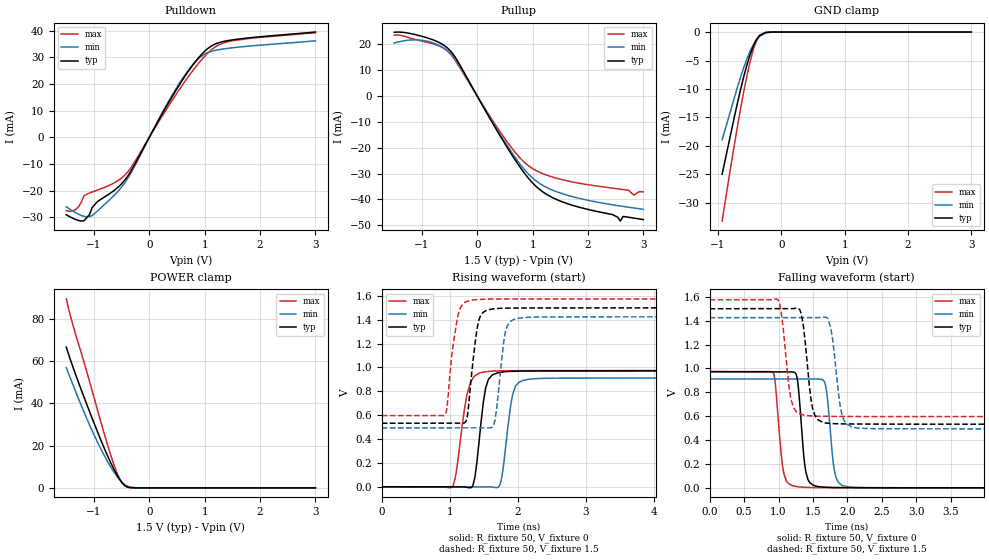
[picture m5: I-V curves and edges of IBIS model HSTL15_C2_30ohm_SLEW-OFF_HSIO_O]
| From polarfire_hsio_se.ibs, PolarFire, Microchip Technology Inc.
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|   Model HSTL15_C2_30ohm_SLEW-OFF_HSIO_O
[Model]   HSTL15_C2_30ohm_SLEW-OFF_HSIO_O
Model_type   Output
Polarity   Non-Inverting
Enable   Active-High
Vmeas =   0.75
Cref =   5p
Rref =   50
Vref =   0.75
|   typ   min   max
C_comp_pullup   1.335e-12   1.335e-12   1.380e-12
C_comp_pulldown  1.335e-12   1.335e-12   1.380e-12
[Temperature Range]  25C   100C   -40C
[Voltage Range]  1.5   1.425   1.575
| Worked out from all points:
|   slope of the pulldown table from 0 to 0.225 V, typ, clamps not added: 26.4 ohm
|   slope of the pullup table from 0 to 0.225 V, typ, clamps not added: 26.4 ohm
|   GND clamp passes 1 mA (typ) near -0.37 V on its own axis
|   POWER clamp passes 1 mA (typ) near -0.43 V on its own axis
|   rising waveform, R_fixture 50, V_fixture 0: 20-80 % time 117ps typ, 120ps min, 143ps max; typ from 0 V to 0.972 V
|   rising waveform, R_fixture 50, V_fixture 1.5: 20-80 % time 111ps typ, 107ps min, 121ps max; typ from 0.533 V to 1.5 V
|   falling waveform, R_fixture 50, V_fixture 0: 20-80 % time 83.1ps typ, 87.6ps min, 88.6ps max; typ from 0.972 V to 0 V
|   falling waveform, R_fixture 50, V_fixture 1.5: 20-80 % time 105ps typ, 112ps min, 108ps max; typ from 1.5 V to 0.533 V
[GND Clamp]
| Voltage   I(typ)   I(min)   I(max)
-935.2mV  -24.96mA   -18.92mA   -33.17mA
-738.3mV  -14.72mA   -11.38mA   -19.54mA
-639.8mV  -9.903mA   -7.788mA   -13.22mA
-590.6mV  -7.7mA     -6.143mA   -10.29mA
-541.4mV  -5.692mA   -4.645mA   -7.577mA
-492.2mV  -3.93mA    -3.33mA    -5.153mA
-443mV    -2.467mA   -2.229mA   -3.103mA
-393.7mV  -1.355mA   -1.366mA   -1.54mA
-344.5mV  -621.9uA   -750.5uA   -567.2uA
-246.1mV  -72.57uA   -154.2uA   -30.93uA
-147.7mV  -5.325uA   -20.63uA   -1.146uA
3V        0A         0A         0A
[POWER Clamp]
| Voltage   I(typ)   I(min)   I(max)
-1.5V     66.64mA    56.9mA     89.46mA
-1.427V   60.81mA    51.96mA    81.57mA
-1.329V   53.43mA    45.4mA     72.34mA
-1.083V   36.31mA    29.95mA    50.59mA
-885.9mV  23.26mA    18.98mA    32.15mA
-738.3mV  14.22mA    11.74mA    18.91mA
-590.6mV  6.331mA    5.649mA    7.47mA
-492.2mV  2.418mA    2.54mA     2.302mA
-443mV    1.134mA    1.422mA    896.4uA
-344.5mV  93.53uA    323uA      39.71uA
-246.1mV  3.484uA    76.21uA    1.36uA
3V        0A         0A         0A
[Pullup]
| Voltage   I(typ)   I(min)   I(max)
-1.5V     24.72mA    20.6mA     23.64mA
-935.2mV  22.77mA    21.42mA    21mA
-492.2mV  17.69mA    16.75mA    16.47mA
609.4mV   -22.23mA   -21.4mA    -19.75mA
890.6mV   -30.94mA   -29.43mA   -26.4mA
1.172V    -36.92mA   -34.44mA   -29.95mA
1.746V    -42.48mA   -39.12mA   -33.38mA
2.435V    -45.85mA   -42.09mA   -35.65mA
2.583V    -48.4mA    -42.58mA   -36.06mA
2.632V    -46.65mA   -42.73mA   -36.2mA
2.829V    -47.27mA   -43.35mA   -38.35mA
3V        -47.83mA   -43.86mA   -37.12mA
[Pulldown]
| Voltage   I(typ)   I(min)   I(max)
-1.5V     -29.1mA    -26.11mA   -27.59mA
-1.329V   -30.88mA   -28.35mA   -27.03mA
-1.23V    -31.45mA   -29.34mA   -24.49mA
-1.083V   -29.08mA   -29.8mA    -20.97mA
-935.2mV  -24.11mA   -27.7mA    -19.8mA
-590.6mV  -19.21mA   -20.85mA   -16.61mA
-344.5mV  -13.14mA   -13.83mA   -11.81mA
562.5mV   20.33mA    20.9mA     18.56mA
843.8mV   28.69mA    28.63mA    26.59mA
1.078V    33.68mA    31.99mA    32.03mA
1.5V      36.55mA    33.59mA    36.2mA
3V        39.5mA     36.21mA    39.23mA
[Ramp]
dV/dt_r   0.583141/0.116851n  0.547234/0.119678n  0.584778/0.143443n
dV/dt_f   0.580324/0.105261n  0.5588/0.111658n  0.587212/0.107647n
R_load = 50
[Rising Waveform]
R_fixture = 50
V_fixture = 0
V_fixture_min = 0
V_fixture_max = 0
| Time   V(typ)   V(min)   V(max)
0s        1.583uV    1.672uV    2.452uV
1.032ns   -626.1uV   -570.8uV   -4.18mV
1.252ns   -4.816mV   -692.8uV   772.9mV
1.314ns   -7.293mV   -727.2uV   886.8mV
1.369ns   82.19mV    -757.7uV   931mV
1.523ns   816.3mV    -843.2uV   964.2mV
1.735ns   958.4mV    15.77mV    971.7mV
1.922ns   967.9mV    770.4mV    973mV
2.147ns   970.2mV    900mV      973.6mV
10ns      971.9mV    912.1mV    974.6mV
[Rising Waveform]
R_fixture = 50
V_fixture = 1.5
V_fixture_min = 1.425
V_fixture_max = 1.575
| Time   V(typ)   V(min)   V(max)
0s        532.8mV    493.6mV    596.3mV
929ps     533.3mV    494.1mV    604.2mV
1.122ns   533.4mV    494.1mV    1.442V
1.248ns   568.1mV    494.2mV    1.552V
1.309ns   879.4mV    494.2mV    1.563V
1.448ns   1.43V      494.3mV    1.571V
1.65ns    1.492V     528.2mV    1.573V
1.815ns   1.497V     1.296V     1.574V
2.024ns   1.498V     1.414V     1.574V
10ns      1.5V       1.425V     1.575V
[Falling Waveform]
R_fixture = 50
V_fixture = 0
V_fixture_min = 0
V_fixture_max = 0
| Time   V(typ)   V(min)   V(max)
0s        971.9mV    912.1mV    974.7mV
924ps     971.2mV    911.5mV    961.1mV
1.078ns   971.1mV    911.4mV    117.9mV
1.26ns    943.6mV    911.3mV    10.78mV
1.396ns   135.9mV    911.2mV    4.517mV
1.577ns   10.8mV     911.1mV    2.071mV
1.698ns   5.016mV    807.1mV    1.534mV
1.834ns   2.412mV    88.43mV    1.28mV
2.013ns   1.487mV    8.407mV    945.2uV
10ns      2.616uV    2.733uV    3.343uV
[Falling Waveform]
R_fixture = 50
V_fixture = 1.5
V_fixture_min = 1.425
V_fixture_max = 1.575
| Time   V(typ)   V(min)   V(max)
0s        1.5V       1.425V     1.575V
994ps     1.501V     1.426V     1.574V
1.18ns    1.501V     1.426V     742.4mV
1.308ns   1.492V     1.426V     620.2mV
1.381ns   1.253V     1.426V     608.3mV
1.532ns   600.6mV    1.426V     600.8mV
1.716ns   541.4mV    1.417V     599mV
1.915ns   535.7mV    628.6mV    598.1mV
2.07ns    535mV      507.8mV    597.7mV
10ns      532.8mV    493.6mV    596.3mV
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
